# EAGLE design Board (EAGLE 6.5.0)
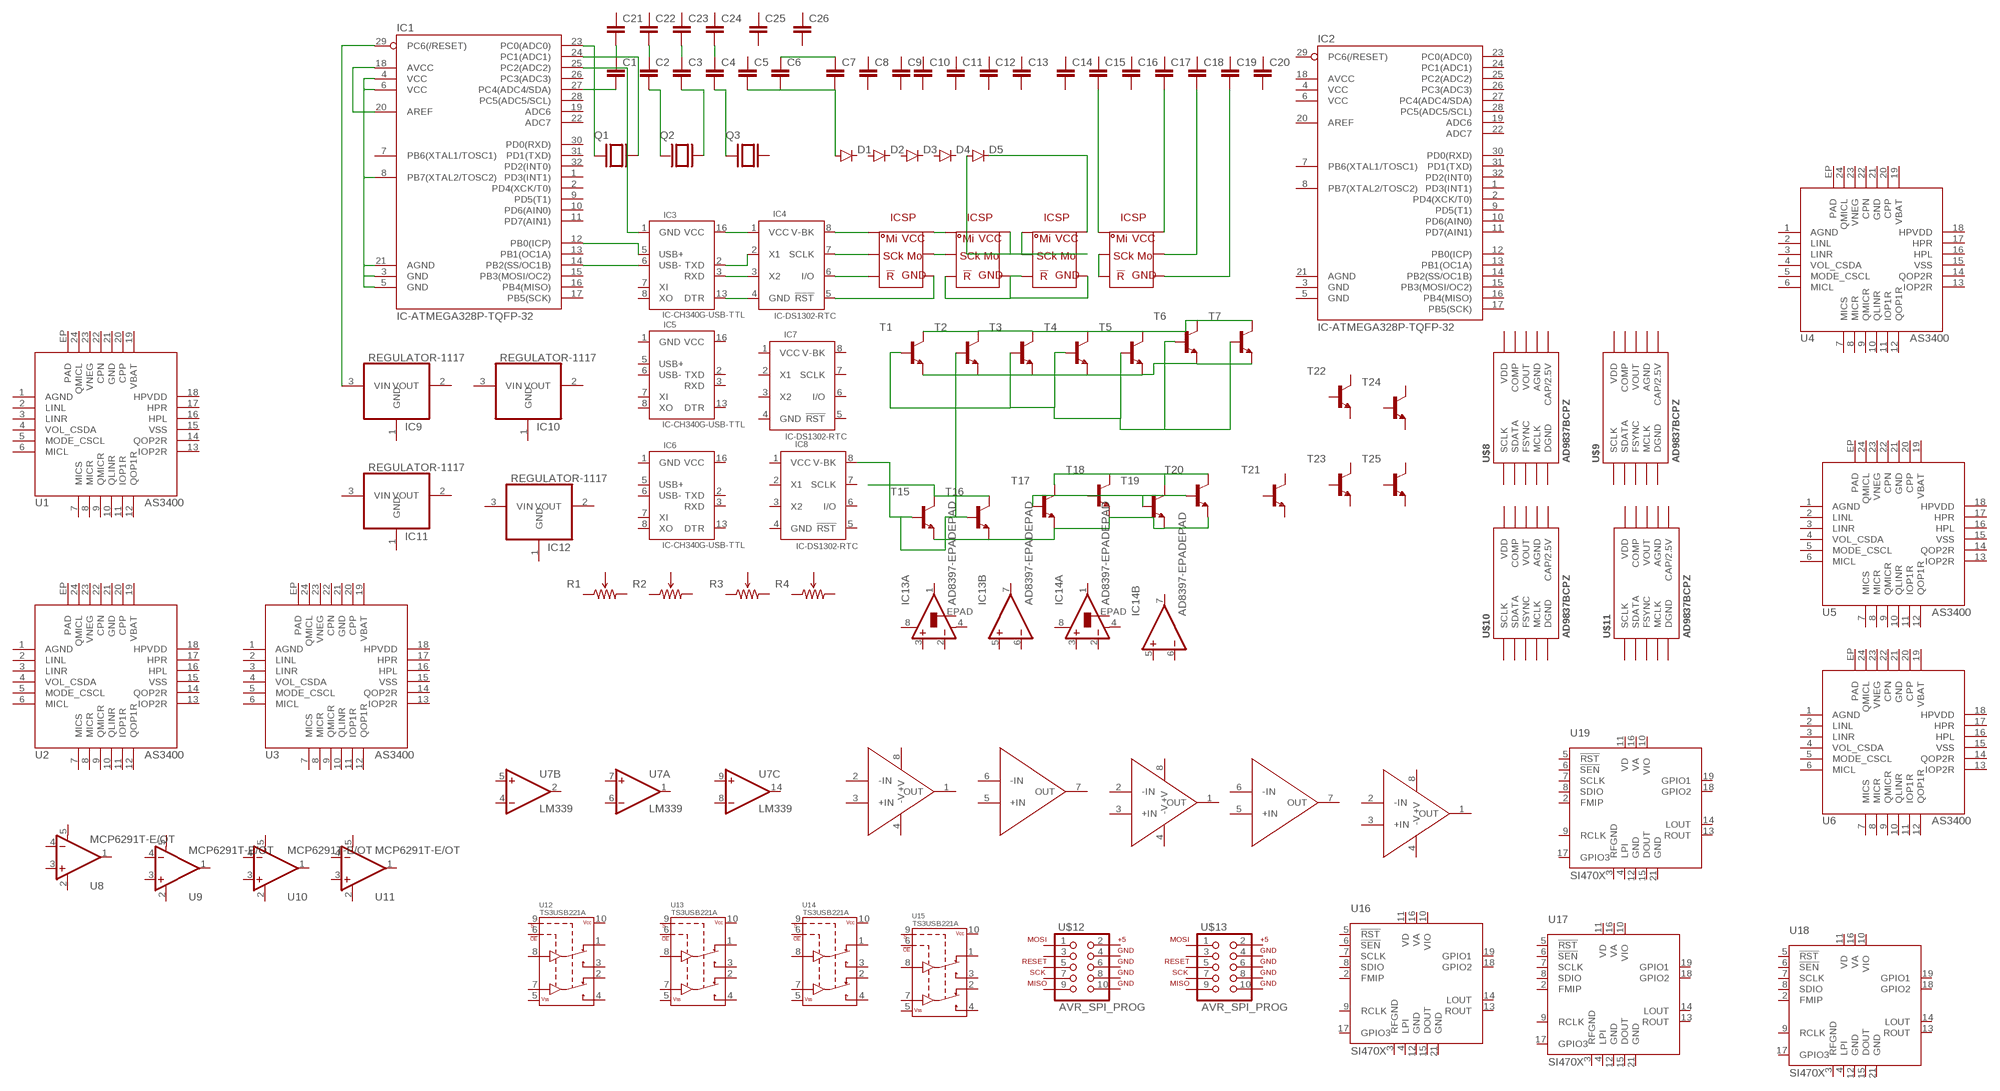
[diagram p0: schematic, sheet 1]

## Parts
C1  CAP-SMD-0603  [0603]
C2  CAP-SMD-0603  [0603]
C3  CAP-SMD-0603  [0603]
C4  CAP-SMD-0603  [0603]
C5  CAP-SMD-0603  [0603]
C6  CAP-SMD-0603  [0603]
C7  CAP-SMD-0805  [0805]
C8  CAP-SMD-0805  [0805]
C9  CAP-SMD-0805  [0805]
C10  CAP-SMD-0805  [0805]
C11  CAP-SMD-0805  [0805]
C12  CAP-SMD-0805  [0805]
C13  CAP-SMD-0805  [0805]
C14  CAP-SMD-1206  [1206]
C15  CAP-SMD-1206  [1206]
C16  CAP-SMD-1206  [1206]
C17  CAP-SMD-1206  [1206]
C18  CAP-SMD-1206  [1206]
C19  CAP-SMD-1206  [1206]
C20  CAP-SMD-1206  [1206]
C21  CAP-SMD-0603  [0603]
C22  CAP-SMD-0603  [0603]
C23  CAP-SMD-0603  [0603]
C24  CAP-SMD-0603  [0603]
C25  CAP-SMD-0603  [0603]
C26  CAP-SMD-0603  [0603]
D1  DIODE-SMA-4MM  [DIODE-SMA]
D2  DIODE-SMA-4MM  [DIODE-SMA]
D3  DIODE-SMA-4MM  [DIODE-SMA]
D4  DIODE-SMA-4MM  [DIODE-SMA]
D5  DIODE-SMA-4MM  [DIODE-SMA]
IC1  IC-ATMEGA328P-TQFP-32  [TQFP32-08MM]
IC2  IC-ATMEGA328P-TQFP-32  [TQFP32-08MM]
IC3  IC-CH340G-USB-TTL  [SOP-16]
IC4  IC-DS1302-RTC  [SOP-08]
IC5  IC-CH340G-USB-TTL  [SOP-16]
IC6  IC-CH340G-USB-TTL  [SOP-16]
IC7  IC-DS1302-RTC  [SOP-08]
IC8  IC-DS1302-RTC  [SOP-08]
IC9  REGULATOR-1117  [SOT-223]
IC10  REGULATOR-1117  [SOT-223]
IC11  REGULATOR-1117  [SOT-223]
IC12  REGULATOR-1117  [SOT-223]
IC13  AD8397-EPADEPAD  [SO08-EPAD]
IC14  AD8397-EPADEPAD  [SO08-EPAD]
Q1  CRYSTAL-5032  [CRYSTAL-5032]
Q2  CRYSTAL-5032  [CRYSTAL-5032]
Q3  CRYSTAL-5032  [CRYSTAL-5032]
R1  POTENTIOMETER-3MM-SMD  [POT-3MM-SMD]
R2  POTENTIOMETER-3MM-SMD  [POT-3MM-SMD]
R3  POTENTIOMETER-3MM-SMD  [POT-3MM-SMD]
R4  POTENTIOMETER-3MM-SMD  [POT-3MM-SMD]
T1  NPN-2SD882-D882-0.5W  [SOT-89]
T2  NPN-2SD882-D882-0.5W  [SOT-89]
T3  NPN-2SD882-D882-0.5W  [SOT-89]
T4  NPN-2SD882-D882-0.5W  [SOT-89]
T5  NPN-2SD882-D882-0.5W  [SOT-89]
T6  NPN-2SD882-D882-0.5W  [SOT-89]
T7  NPN-2SD882-D882-0.5W  [SOT-89]
T15  NPN-S9018-J8-0.2W  [SOT-23]
T16  NPN-S9018-J8-0.2W  [SOT-23]
T17  NPN-S9018-J8-0.2W  [SOT-23]
T18  NPN-S9018-J8-0.2W  [SOT-23]
T19  NPN-S9018-J8-0.2W  [SOT-23]
T20  NPN-S9018-J8-0.2W  [SOT-23]
T21  NPN-S9018-J8-0.2W  [SOT-23]
T22  NPN-TO-92  [TO-92]
T23  NPN-TO-92  [TO-92]
T24  NPN-TO-92  [TO-92]
T25  NPN-TO-92  [TO-92]
U1  AS3400  [QFN-24_ALT2]
U2  AS3400  [QFN-24_ALT2]
U3  AS3400  [QFN-24_ALT2]
U4  AS3400  [QFN-24_ALT2]
U5  AS3400  [QFN-24_ALT2]
U6  AS3400  [QFN-24_ALT2]
U7  LM339  [TSSOP-14]
U8  MCP6291T-E/OT  [SOT23-5]
U9  MCP6291T-E/OT  [SOT23-5]
U10  MCP6291T-E/OT  [SOT23-5]
U11  MCP6291T-E/OT  [SOT23-5]
U12  TS3USB221A  [QFN-10-RSE]
U13  TS3USB221A  [QFN-10-RSE]
U14  TS3USB221A  [QFN-10-RSE]
U15  TS3USB221A  [QFN-10-RSE]
U16  SI470X  [SI470X]
U17  SI470X  [SI470X]
U18  SI470X  [SI470X]
U19  SI470X  [SI470X]
U$1  ISCP-6PINS  [ISCP]
U$2  ISCP-6PINS  [ISCP]
U$3  ISCP-6PINS  [ISCP]
U$4  ISCP-6PINS  [ISCP]
U$5  LTC6244  [MSOP8]
U$6  LTC6244  [MSOP8]
U$7  LTC6244  [MSOP8]
U$8  AD9837BCPZ  AD9837  [AD9837]
U$9  AD9837BCPZ  AD9837  [AD9837]
U$10  AD9837BCPZ  AD9837  [AD9837]
U$11  AD9837BCPZ  AD9837  [AD9837]
U$12  AVR_SPI_PROG  [AVR_ICSP]
U$13  AVR_SPI_PROG  [AVR_ICSP]

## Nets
N$27: IC1.29(PC6(/RESET)) IC9.3(VIN)
N$28: IC1.18(AVCC) IC1.20(AREF)
N$29: IC1.6(VCC) IC1.8(PB7(XTAL2/TOSC2))
N$30: IC1.3(GND) IC1.4(VCC) IC1.5(GND) IC1.21(AGND)
N$31: IC1.23(PC0(ADC0)) Q1.1
N$32: C21.2 IC1.24(PC1(ADC1)) Q1.2
N$33: C6.1 C7.1
N$34: C5.2 D1.A
N$35: C4.2 Q3.1
N$36: C3.2 Q2.2
N$37: C2.2 Q2.1
N$38: C4.1 C24.2
N$39: C3.1 C23.2
N$40: C2.1 C22.2
N$41: C1.2 IC1.27(PC4(ADC4/SDA))
N$42: IC1.25(PC2(ADC2)) IC3.1(GND)
N$43: IC1.12(PB0(ICP)) IC3.5(USB+)
N$44: IC1.14(PB2(SS/OC1B)) IC3.6(USB-)
N$45: IC3.16(VCC) IC4.1(VCC)
N$46: IC3.3(RXD) IC4.3(X2)
N$47: IC3.2(TXD) IC4.2(X1)
N$48: IC3.13(DTR) IC4.4(GND)
N$49: IC4.8(V-BK) U$1.P$1
N$50: IC4.7(SCLK) U$1.P$2
N$51: IC4.6(I/O) U$1.P$3
N$52: IC4.5(!RST) U$1.P$4
N$53: U$1.P$5 U$2.P$2
N$54: U$1.P$6 U$2.P$1
N$55: U$2.P$3 U$2.P$4 U$3.P$3 U$3.P$4
N$56: U$2.P$5 U$2.P$6
N$57: U$3.P$1 U$3.P$2
N$59: D5.C U$3.P$6
N$60: C15.2 U$4.P$1
N$61: D5.A U$3.P$5
N$62: U$4.P$2 U$4.P$3
N$63: C17.2 U$4.P$6
N$64: C18.2 U$4.P$5
N$65: C19.2 U$4.P$4
N$66: IC8.8(V-BK) T15.1(B) T16.1(B)
N$67: T15.3(C) T16.3(C)
N$68: T2.1(B)
N$69: T1.1(B) T3.1(B) T4.1(B) T5.1(B) T6.1(B) T7.1(B)
N$74: T1.2(C) T2.2(C) T3.2(C) T4.2(C) T5.2(C) T6.2(C) T7.2(C)
N$75: T1.3(E) T2.3(E) T3.3(E) T4.3(E) T5.3(E) T6.3(E) T7.3(E)
N$78: T15.2(E) T16.2(E) T17.2(E) T18.2(E) T19.2(E) T20.2(E)
N$81: T17.3(C) T18.3(C) T19.3(C) T20.3(C)
N$82: T17.1(B) T18.1(B) T19.1(B) T20.1(B)
Unconnected: C1.1 C5.1 C6.2 C7.2 C8.1 C8.2 C9.1 C9.2 C10.1 C10.2 C11.1 C11.2 C12.1 C12.2 C13.1 C13.2 C14.1 C14.2 C15.1 C16.1 C16.2 C17.1 C18.1 C19.1 C20.1 C20.2 C21.1 C22.1 C23.1 C24.1 C25.1 C25.2 C26.1 C26.2 D1.C D2.A D2.C D3.A D3.C D4.A D4.C IC1.1(PD3(INT1)) IC1.2(PD4(XCK/T0)) IC1.7(PB6(XTAL1/TOSC1)) IC1.9(PD5(T1)) IC1.10(PD6(AIN0)) IC1.11(PD7(AIN1)) IC1.13(PB1(OC1A)) IC1.15(PB3(MOSI/OC2)) IC1.16(PB4(MISO)) IC1.17(PB5(SCK)) IC1.19(ADC6) IC1.22(ADC7) IC1.26(PC3(ADC3)) IC1.28(PC5(ADC5/SCL)) IC1.30(PD0(RXD)) IC1.31(PD1(TXD)) IC1.32(PD2(INT0)) IC2.1(PD3(INT1)) IC2.2(PD4(XCK/T0)) IC2.3(GND) IC2.4(VCC) IC2.5(GND) IC2.6(VCC) IC2.7(PB6(XTAL1/TOSC1)) IC2.8(PB7(XTAL2/TOSC2)) IC2.9(PD5(T1)) IC2.10(PD6(AIN0)) IC2.11(PD7(AIN1)) IC2.12(PB0(ICP)) IC2.13(PB1(OC1A)) IC2.14(PB2(SS/OC1B)) IC2.15(PB3(MOSI/OC2)) IC2.16(PB4(MISO)) IC2.17(PB5(SCK)) IC2.18(AVCC) IC2.19(ADC6) IC2.20(AREF) IC2.21(AGND) IC2.22(ADC7) IC2.23(PC0(ADC0)) IC2.24(PC1(ADC1)) IC2.25(PC2(ADC2)) IC2.26(PC3(ADC3)) IC2.27(PC4(ADC4/SDA)) IC2.28(PC5(ADC5/SCL)) IC2.29(PC6(/RESET)) IC2.30(PD0(RXD)) IC2.31(PD1(TXD)) IC2.32(PD2(INT0)) IC3.7(XI) IC3.8(XO) IC5.1(GND) IC5.2(TXD) IC5.3(RXD) IC5.5(USB+) IC5.6(USB-) IC5.7(XI) IC5.8(XO) IC5.13(DTR) IC5.16(VCC) IC6.1(GND) IC6.2(TXD) IC6.3(RXD) IC6.5(USB+) IC6.6(USB-) IC6.7(XI) IC6.8(XO) IC6.13(DTR) IC6.16(VCC) IC7.1(VCC) IC7.2(X1) IC7.3(X2) IC7.4(GND) IC7.5(!RST) IC7.6(I/O) IC7.7(SCLK) IC7.8(V-BK) IC8.1(VCC) IC8.2(X1) IC8.3(X2) IC8.4(GND) IC8.5(!RST) IC8.6(I/O) IC8.7(SCLK) IC9.2(VOUT) IC10.2(VOUT) IC10.3(VIN) IC11.2(VOUT) IC11.3(VIN) IC12.2(VOUT) IC12.3(VIN) IC13.1(A:OUT) IC13.2(A:-IN) IC13.3(A:+IN) IC13.5(B:+IN) IC13.6(B:-IN) IC13.7(B:OUT) IC13.EPAD(A:EPAD) IC14.1(A:OUT) IC14.2(A:-IN) IC14.3(A:+IN) IC14.5(B:+IN) IC14.6(B:-IN) IC14.7(B:OUT) IC14.EPAD(A:EPAD) Q3.2 R1.1(CCW) R1.2(WIPER) R1.3(CW) R2.1(CCW) R2.2(WIPER) R2.3(CW) R3.1(CCW) R3.2(WIPER) R3.3(CW) R4.1(CCW) R4.2(WIPER) R4.3(CW) T21.1(B) T21.2(E) T21.3(C) T22.1(E) T22.2(B) T22.3(C) T23.1(E) T23.2(B) T23.3(C) T24.1(E) T24.2(B) T24.3(C) T25.1(E) T25.2(B) T25.3(C) U1.1(AGND) U1.2(LINL) U1.3(LINR) U1.4(VOL_CSDA) U1.5(MODE_CSCL) U1.6(MICL) U1.7(MICS) U1.8(MICR) U1.9(QMICR) U1.10(QLINR) U1.11(IOP1R) U1.12(QOP1R) U1.13(IOP2R) U1.14(QOP2R) U1.15(VSS) U1.16(HPL) U1.17(HPR) U1.18(HPVDD) U1.19(VBAT) U1.20(CPP) U1.21(GND) U1.22(CPN) U1.23(VNEG) U1.24(QMICL) U1.EP(PAD) U2.1(AGND) U2.2(LINL) U2.3(LINR) U2.4(VOL_CSDA) U2.5(MODE_CSCL) U2.6(MICL) U2.7(MICS) U2.8(MICR) U2.9(QMICR) U2.10(QLINR) U2.11(IOP1R) U2.12(QOP1R) U2.13(IOP2R) U2.14(QOP2R) U2.15(VSS) U2.16(HPL) U2.17(HPR) U2.18(HPVDD) U2.19(VBAT) U2.20(CPP) U2.21(GND) U2.22(CPN) U2.23(VNEG) U2.24(QMICL) U2.EP(PAD) U3.1(AGND) U3.2(LINL) U3.3(LINR) U3.4(VOL_CSDA) U3.5(MODE_CSCL) U3.6(MICL) U3.7(MICS) U3.8(MICR) U3.9(QMICR) U3.10(QLINR) U3.11(IOP1R) U3.12(QOP1R) U3.13(IOP2R) U3.14(QOP2R) U3.15(VSS) U3.16(HPL) U3.17(HPR) U3.18(HPVDD) U3.19(VBAT) U3.20(CPP) U3.21(GND) U3.22(CPN) U3.23(VNEG) U3.24(QMICL) U3.EP(PAD) U4.1(AGND) U4.2(LINL) U4.3(LINR) U4.4(VOL_CSDA) U4.5(MODE_CSCL) U4.6(MICL) U4.7(MICS) U4.8(MICR) U4.9(QMICR) U4.10(QLINR) U4.11(IOP1R) U4.12(QOP1R) U4.13(IOP2R) U4.14(QOP2R) U4.15(VSS) U4.16(HPL) U4.17(HPR) U4.18(HPVDD) U4.19(VBAT) U4.20(CPP) U4.21(GND) U4.22(CPN) U4.23(VNEG) U4.24(QMICL) U4.EP(PAD) U5.1(AGND) U5.2(LINL) U5.3(LINR) U5.4(VOL_CSDA) U5.5(MODE_CSCL) U5.6(MICL) U5.7(MICS) U5.8(MICR) U5.9(QMICR) U5.10(QLINR) U5.11(IOP1R) U5.12(QOP1R) U5.13(IOP2R) U5.14(QOP2R) U5.15(VSS) U5.16(HPL) U5.17(HPR) U5.18(HPVDD) U5.19(VBAT) U5.20(CPP) U5.21(GND) U5.22(CPN) U5.23(VNEG) U5.24(QMICL) U5.EP(PAD) U6.1(AGND) U6.2(LINL) U6.3(LINR) U6.4(VOL_CSDA) U6.5(MODE_CSCL) U6.6(MICL) U6.7(MICS) U6.8(MICR) U6.9(QMICR) U6.10(QLINR) U6.11(IOP1R) U6.12(QOP1R) U6.13(IOP2R) U6.14(QOP2R) U6.15(VSS) U6.16(HPL) U6.17(HPR) U6.18(HPVDD) U6.19(VBAT) U6.20(CPP) U6.21(GND) U6.22(CPN) U6.23(VNEG) U6.24(QMICL) U6.EP(PAD) U7.1(A:OUT) U7.2(B:OUT) U7.4(B:-IN) U7.5(B:+IN) U7.6(A:-IN) U7.7(A:+IN) U7.8(C:-IN) U7.9(C:+IN) U7.10(D:-IN) U7.11(D:+IN) U7.13(D:OUT) U7.14(C:OUT) U8.1(OUT) U8.3(+IN) U8.4(-IN) U9.1(OUT) U9.3(+IN) U9.4(-IN) U10.1(OUT) U10.3(+IN) U10.4(-IN) U11.1(OUT) U11.3(+IN) U11.4(-IN) U12.1(1D+) U12.2(1D-) U12.3(2D+) U12.4(2D-) U12.5(VSS) U12.6(!OE) U12.7(D-) U12.8(D+) U12.9(S) U12.10(VCC) U13.1(1D+) U13.2(1D-) U13.3(2D+) U13.4(2D-) U13.5(VSS) U13.6(!OE) U13.7(D-) U13.8(D+) U13.9(S) U13.10(VCC) U14.1(1D+) U14.2(1D-) U14.3(2D+) U14.4(2D-) U14.5(VSS) U14.6(!OE) U14.7(D-) U14.8(D+) U14.9(S) U14.10(VCC) U15.1(1D+) U15.2(1D-) U15.3(2D+) U15.4(2D-) U15.5(VSS) U15.6(!OE) U15.7(D-) U15.8(D+) U15.9(S) U15.10(VCC) U16.2(FMIP) U16.3(RFGND) U16.4(LPI) U16.5(!RST) U16.6(!SEN) U16.7(SCLK) U16.8(SDIO) U16.9(RCLK) U16.10(VIO) U16.11(VD) U16.12(GND) U16.13(ROUT) U16.14(LOUT) U16.15(DOUT) U16.16(VA) U16.17(GPIO3) U16.18(GPIO2) U16.19(GPIO1) U16.21(GND) U17.2(FMIP) U17.3(RFGND) U17.4(LPI) U17.5(!RST) U17.6(!SEN) U17.7(SCLK) U17.8(SDIO) U17.9(RCLK) U17.10(VIO) U17.11(VD) U17.12(GND) U17.13(ROUT) U17.14(LOUT) U17.15(DOUT) U17.16(VA) U17.17(GPIO3) U17.18(GPIO2) U17.19(GPIO1) U17.21(GND) U18.2(FMIP) U18.3(RFGND) U18.4(LPI) U18.5(!RST) U18.6(!SEN) U18.7(SCLK) U18.8(SDIO) U18.9(RCLK) U18.10(VIO) U18.11(VD) U18.12(GND) U18.13(ROUT) U18.14(LOUT) U18.15(DOUT) U18.16(VA) U18.17(GPIO3) U18.18(GPIO2) U18.19(GPIO1) U18.21(GND) U19.2(FMIP) U19.3(RFGND) U19.4(LPI) U19.5(!RST) U19.6(!SEN) U19.7(SCLK) U19.8(SDIO) U19.9(RCLK) U19.10(VIO) U19.11(VD) U19.12(GND) U19.13(ROUT) U19.14(LOUT) U19.15(DOUT) U19.16(VA) U19.17(GPIO3) U19.18(GPIO2) U19.19(GPIO1) U19.21(GND) U$5.1(OUT) U$5.2(-IN) U$5.3(+IN) U$5.4(-V) U$5.5(+IN) U$5.6(-IN) U$5.7(OUT) U$5.8(+V) U$6.1(OUT) U$6.2(-IN) U$6.3(+IN) U$6.4(-V) U$6.5(+IN) U$6.6(-IN) U$6.7(OUT) U$6.8(+V) U$7.1(OUT) U$7.2(-IN) U$7.3(+IN) U$7.4(-V) U$7.5(+IN) U$7.6(-IN) U$7.7(OUT) U$7.8(+V) U$8.P$0(DGND) U$8.P$1(COMP) U$8.P$2(VDD) U$8.P$3(CAP/2.5V) U$8.P$4(DGND) U$8.P$5(MCLK) U$8.P$6(SDATA) U$8.P$7(SCLK) U$8.P$8(FSYNC) U$8.P$9(AGND) U$8.P$10(VOUT) U$9.P$0(DGND) U$9.P$1(COMP) U$9.P$2(VDD) U$9.P$3(CAP/2.5V) U$9.P$4(DGND) U$9.P$5(MCLK) U$9.P$6(SDATA) U$9.P$7(SCLK) U$9.P$8(FSYNC) U$9.P$9(AGND) U$9.P$10(VOUT) U$10.P$0(DGND) U$10.P$1(COMP) U$10.P$2(VDD) U$10.P$3(CAP/2.5V) U$10.P$4(DGND) U$10.P$5(MCLK) U$10.P$6(SDATA) U$10.P$7(SCLK) U$10.P$8(FSYNC) U$10.P$9(AGND) U$10.P$10(VOUT) U$11.P$0(DGND) U$11.P$1(COMP) U$11.P$2(VDD) U$11.P$3(CAP/2.5V) U$11.P$4(DGND) U$11.P$5(MCLK) U$11.P$6(SDATA) U$11.P$7(SCLK) U$11.P$8(FSYNC) U$11.P$9(AGND) U$11.P$10(VOUT) U$12.1 U$12.2 U$12.3 U$12.4 U$12.5 U$12.6 U$12.7 U$12.8 U$12.9 U$12.10 U$13.1 U$13.2 U$13.3 U$13.4 U$13.5 U$13.6 U$13.7 U$13.8 U$13.9 U$13.10

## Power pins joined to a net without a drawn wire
GND: IC9.1(GND) IC10.1(GND) IC11.1(GND) IC12.1(GND) U7.12(P:GND)
V+: IC13.8(A:V+) IC14.8(A:V+) U8.5(V+) U9.5(V+) U10.5(V+) U11.5(V+)
V-: IC13.4(A:V-) IC14.4(A:V-) U8.2(V-) U9.2(V-) U10.2(V-) U11.2(V-)
VCC: U7.3(P:VCC)

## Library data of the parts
C1-C26 = - Jins eagle lbr:CAP-SMD
D1-D5 = - Jins eagle lbr:DIODE: Diode
IC1 IC2 = - Jins eagle lbr:IC-ATMEGA328P-TQFP-32
IC3 IC5 IC6 = - Jins eagle lbr:IC-CH340G
IC4 IC7 IC8 = - Jins eagle lbr:IC-DS1302
IC9-IC12 = - Jins eagle lbr:REGULATOR: 800mA and 1A Low Dropout (LDO) Positive Regulator 1.8V, 2.5V, 2.85V, 3.3V, 5V, and Adj; MPN: REG1117; OC_FARNELL: 1097566; OC_NEWARK: 14P6981
IC13 IC14 = SparkFun-AnalogIC:AD8397-EPAD: Rail-to-rail high current output op-amp
Q1-Q3 = - Jins eagle lbr:CRYSTAL: CRYSTAL
R1-R4 = - Jins eagle lbr:POTENTIOMETER
T1-T7 T15-T25 = - Jins eagle lbr:NPN
U1-U6 = SparkFun-AnalogIC:AS3400: Active noise cancellation chip. Stereo in, stereo out, two microphones. Single alkaline cell power. QFN-24 w/exposed pad.
U7 = SparkFun-AnalogIC:LM339: Based on information from the SLCS006N datasheet from TI (www.ti.com). Change Log DateAuthorChange July 16, 2008nick@scantool.netDevice created.; DESC: IC, Quad Comparator; MANUF: Texas Instruments; PARTNUM: LM339PWR; SUPPLIER: Digikey:296-6607-1-ND; VALSTAT: PARTNUM
U8-U11 = SparkFun-AnalogIC:MCP6291: Rail to rail OpAmp with 10MHz GBP; PROD_ID: IC-11991
U12-U15 = SparkFun-AnalogIC:TS3USB221A: DPDT Analog Mux Vcc 2.5 to 3.3V Passes up to 5.5V at 3.3V supply 900MHz BW, 6&#8486; switch resistance; PROD_ID: IC-12115
U16-U19 = SparkFun-RF:SI470X: FM receiver IC. Tested with Si4703. You really only need SEN, RST, SCLK, and SDIO to get a full FM radio working. Antenna comes from headphone jack. See BOB-10344.
U$1-U$4 = - Jins eagle lbr:ISCP
U$5-U$7 = SparkFun-AnalogIC:LTC6244: Low-noise, high-speed rail-to-rail CMOS op-amp
U$8-U$11 = SparkFun-AnalogIC:AD9837: Programmable waveform generator, sine, triangular, and square wave outputs.; PROD_ID: IC-11223
U$12 U$13 = SparkFun-Connectors:AVR_SPI_PROG: AVR 10-pin ICSP Header This is the standard AVR In Circuit Serial Programming header. Minimal, but includes pin one indicator. Works with standard Olimex programmers. Also look for the 6-pin reduced version. Spark Fun Electronics SKU: PRT-00778

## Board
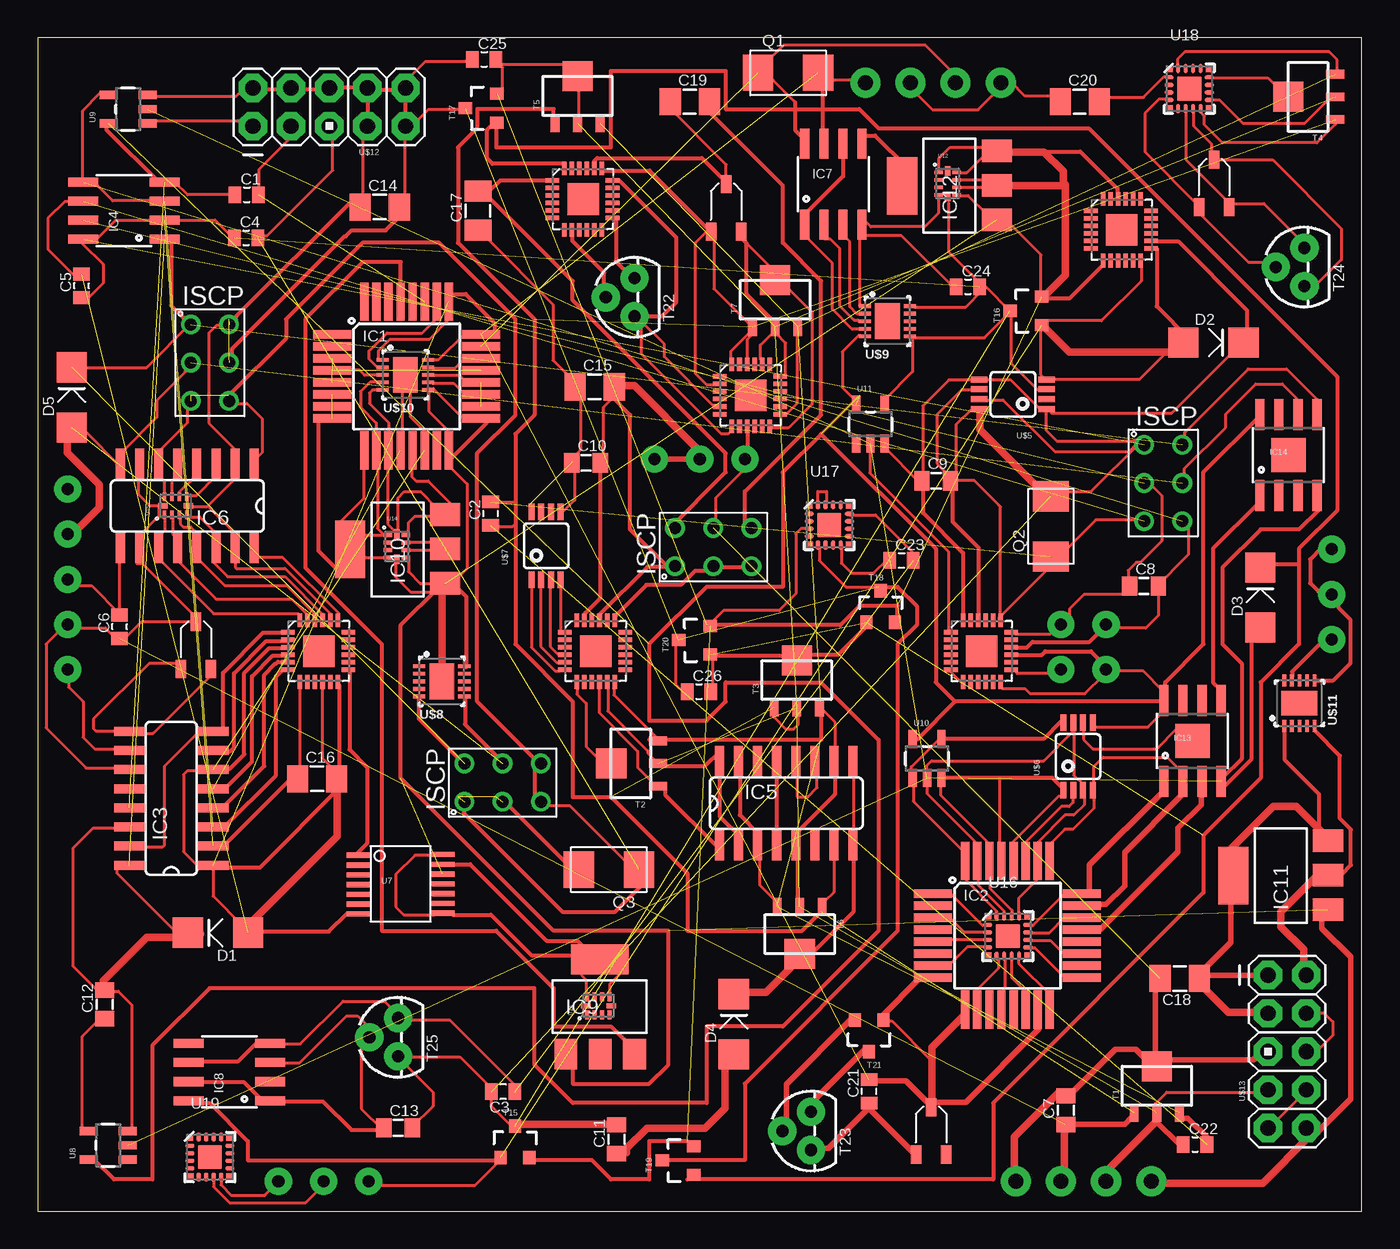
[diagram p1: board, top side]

Size 88 x 78 mm. Coordinates in mm from the lower left corner, seen from the top.
Outline: 0,0 88,0 88,78 0,78 0,0
Copper layers (1*16): Top 0.035mm / dielectric 1.5mm / Bottom 0.035mm
Design rules "default": minimum track width 10mil, minimum drill 24mil, track to track 8mil, track to pad 8mil, pad to pad 8mil, via to via 8mil, smd to smd 8mil, copper to edge 40mil, drill to drill 8mil, minimum pad ring 10mil, minimum via ring 8mil, stop-mask expansion 4mil, vias tented up to drill 0mil, thermal gap 10mil

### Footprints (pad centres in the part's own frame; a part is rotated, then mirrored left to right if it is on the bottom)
0603 = smd 0.838 x 1.1: 1 -0.781,0; 2 0.781,0
0805 = smd 1.016 x 1.27: 1 -0.95,0; 2 0.95,0
1206 = smd 1.4 x 1.8: 1 -1.3,0; 2 1.3,0
DIODE-SMA = smd 2 x 2: A -2,0; C 2,0
TQFP32-08MM = smd 2.54 x 0.559: 1 -6.502,6.75; 2 -6.502,5.95; 3 -6.502,5.15; 4 -6.502,4.35; 5 -6.502,3.55; 6 -6.502,2.75; 7 -6.502,1.95; 8 -6.502,1.15; 17 3.404,1.15; 18 3.404,1.95; 19 3.404,2.75; 20 3.404,3.55; 21 3.404,4.35; 22 3.404,5.15; 23 3.404,5.95; 24 3.404,6.75 | smd 0.559 x 2.54: 9 -4.35,-0.965; 10 -3.55,-0.965; 11 -2.75,-0.965; 12 -1.95,-0.965; 13 -1.15,-0.965; 14 -0.35,-0.965; 15 0.45,-0.965; 16 1.25,-0.965; 25 1.25,8.915; 26 0.45,8.915; 27 -0.35,8.915; 28 -1.15,8.915; 29 -1.95,8.915; 30 -2.75,8.915; 31 -3.55,8.915; 32 -4.35,8.915
SOP-16 = smd 0.6 x 2: 1 -3.945,-2.76; 2 -2.675,-2.76; 3 -1.405,-2.76; 4 -0.135,-2.76; 5 1.135,-2.76; 6 2.405,-2.76; 7 3.675,-2.76; 8 4.945,-2.76; 9 4.945,2.84; 10 3.675,2.84; 11 2.405,2.84; 12 1.135,2.84; 13 -0.135,2.84; 14 -1.405,2.84; 15 -2.675,2.84; 16 -3.945,2.84
SOP-08 = smd 0.6 x 2: 1 -1.905,-2.7; 2 -0.635,-2.7; 3 0.635,-2.7; 4 1.905,-2.7; 5 1.905,2.7; 6 0.635,2.7; 7 -0.635,2.7; 8 -1.905,2.7
SOT-223 = smd 1.499 x 2.007: 1 -2.261,-3.15; 2 0.025,-3.15; 3 2.311,-3.15 | smd 3.81 x 2.007: 4 0,3.15
SO08-EPAD = smd 0.61 x 2.057: 1 -1.905,-2.692; 2 -0.635,-2.692; 3 0.635,-2.692; 4 1.905,-2.692; 5 1.905,2.692; 6 0.635,2.692; 7 -0.635,2.692; 8 -1.905,2.692 | smd 2.286 x 2.286: EPAD 0,0
CRYSTAL-5032 = smd 2 x 2.4: 1 -2,0; 2 2,0
POT-3MM-SMD = smd 0.7 x 1.2: 1 -1,-1.55; 2 0,1.6; 3 1,-1.55
SOT-89 = smd 0.58 x 1.2: 1 -1.5,-1.8; 2 0,-1.8; 3 1.5,-1.8 | smd 2 x 2: 4 0,1.3
SOT-23 = smd 0.8 x 0.9: 1 -1.315,-0.635; 2 0.585,-0.635; 3 -0.365,1.465
TO-92 = drill 0.813 pad 1.88: 1 -1.27,0; 2 0,1.905; 3 1.27,0
QFN-24_ALT2 = smd 0.9 x 0.3: 1 -2.05,1.25; 2 -2.05,0.75; 3 -2.05,0.25; 4 -2.05,-0.25; 5 -2.05,-0.75; 6 -2.05,-1.25; 13 1.95,-1.25; 14 1.95,-0.75; 15 1.95,-0.25; 16 1.95,0.25; 17 1.95,0.75; 18 1.95,1.25 | smd 0.3 x 0.9: 7 -1.25,-2.05; 8 -0.75,-2.05; 9 -0.25,-2.05; 10 0.25,-2.05; 11 0.75,-2.05; 12 1.25,-2.05; 19 1.25,2.05; 20 0.75,2.05; 21 0.25,2.05; 22 -0.25,2.05; 23 -0.75,2.05; 24 -1.25,2.05 | smd 2.1 x 2.1: EP 0,0
TSSOP-14 = smd 1.6 x 0.35: 1 -2.8,1.9; 2 -2.8,1.25; 3 -2.8,0.6; 4 -2.8,-0.05; 5 -2.8,-0.7; 6 -2.8,-1.35; 7 -2.8,-2; 8 2.8,-1.95; 9 2.8,-1.3; 10 2.8,-0.65; 11 2.8,0; 12 2.8,0.65; 13 2.8,1.3; 14 2.8,1.95
SOT23-5 = smd 0.55 x 1.2: 1 -0.95,-1.3; 2 0,-1.3; 3 0.95,-1.3; 4 0.95,1.3; 5 -0.95,1.3
QFN-10-RSE = smd 0.58 x 0.25: 1 -0.6,0.75; 2 -0.6,0.25; 3 -0.6,-0.25; 4 -0.6,-0.75; 6 0.6,-0.75; 7 0.6,-0.25; 8 0.6,0.25; 9 0.6,0.75 | smd 0.35 x 0.63: 5 0,-0.85; 10 0,0.85
SI470X = smd 0.34 x 0.34: 1 -1.275,1.265; 6 -1.265,-1.265; 11 1.265,-1.265; 16 1.265,1.265 | smd 0.61 x 0.28: 2 -1.335,0.75; 3 -1.335,0.25; 4 -1.335,-0.25; 5 -1.335,-0.75; 12 1.335,-0.75; 13 1.335,-0.25; 14 1.335,0.25; 15 1.335,0.75 | smd 0.28 x 0.61: 7 -0.75,-1.335; 8 -0.25,-1.335; 9 0.25,-1.335; 10 0.75,-1.335; 17 0.75,1.335; 18 0.25,1.335; 19 -0.25,1.335; 20 -0.75,1.335 | smd 1.6 x 1.6: 21 0,0
ISCP = drill 0.8: P$1 -2.54,2.54; P$2 -2.54,0; P$3 -2.54,-2.54; P$4 0,-2.54; P$5 0,0; P$6 0,2.54
MSOP8 = smd 0.4 x 1.1: 1 -0.975,-2.25; 2 -0.325,-2.25; 3 0.325,-2.25; 4 0.975,-2.25; 5 0.975,2.25; 6 0.325,2.25; 7 -0.325,2.25; 8 -0.975,2.25
AD9837 = smd 1.64 x 2.38: P$0 0,0 | smd 0.8 x 0.25: P$1 -1.5,1; P$2 -1.5,0.5; P$3 -1.5,0; P$4 -1.5,-0.5; P$5 -1.5,-1; P$6 1.5,-1; P$7 1.5,-0.5; P$8 1.5,0; P$9 1.5,0.5; P$10 1.5,1
AVR_ICSP = drill 1.016 pad 1.88 octagon: 1 -1.27,5.08; 2 1.27,5.08; 3 -1.27,2.54; 4 1.27,2.54; 5 -1.27,0; 6 1.27,0; 7 -1.27,-2.54; 8 1.27,-2.54; 9 -1.27,-5.08; 10 1.27,-5.08

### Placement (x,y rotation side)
C1  13.9,67.55 0 top
C2  30.1,46.37 90 top
C3  30.94,7.96 180 top
C4  13.85,64.7 0 top
C5  2.92,61.5 90 top
C6  5.45,38.85 90 top
C7  68.33,6.72 90 top
C8  73.52,41.55 0 top
C9  59.71,48.55 0 top
C10  36.45,49.74 0 top
C11  38.47,4.8 90 top
C12  4.45,13.76 90 top
C13  23.95,5.55 0 top
C14  22.74,66.74 0 top
C15  37.02,54.79 0 top
C16  18.58,28.74 0 top
C17  29.26,66.5 90 top
C18  75.89,15.48 180 top
C19  43.34,73.74 0 top
C20  69.26,73.74 0 top
C21  55.24,7.97 90 top
C22  76.91,4.44 0 top
C23  57.4,43.25 0 top
C24  61.82,61.44 0 top
C25  29.67,76.55 0 top
C26  43.94,34.54 0 top
D1  11.99,18.52 180 top
D2  78.14,57.74 0 top
D3  81.26,40.79 90 top
D4  46.26,12.44 90 top
D5  2.26,54.09 90 top
IC1  26.07,51.54 0 top
IC2  66,14.37 0 top
IC3  8.92,26.95 90 top
IC4  5.74,66.5 90 top
IC5  49.25,27.08 0 top
IC6  10.45,46.92 180 top
IC7  52.88,68.26 0 top
IC8  12.74,9.26 90 top
IC9  37.35,13.6 0 top
IC10  23.92,44 90 top
IC11  82.6,22.31 90 top
IC12  60.6,68.15 90 top
IC13  76.74,31.26 0 top
IC14  83.12,50.26 0 top
Q1  49.87,75.66 0 top
Q2  67.34,45.52 90 top
Q3  37.96,22.71 180 top
R1  10.53,37.58 0 top
R2  59.38,5.33 0 top
R3  45.76,66.66 0 top
R4  78.17,68.29 0 top
T1  74.37,8.34 0 top
T2  39.42,29.76 90 top
T3  50.45,35.3 0 top
T4  84.42,74.06 90 top
T5  35.88,74.12 0 top
T6  50.64,18.42 180 top
T7  49.01,60.58 0 top
T15  32.09,4.21 0 top
T16  66.09,60.21 90 top
T17  29.89,73.67 90 top
T18  56.39,39.77 0 top
T19  42.96,3.75 90 top
T20  44.07,38.32 90 top
T21  54.89,12.08 180 top
T22  39.66,60.75 90 top
T23  51.39,5.34 90 top
T24  84.18,62.75 90 top
T25  23.95,11.57 90 top
U1  36.25,67.26 0 top
U2  37.09,37.23 0 top
U3  62.74,37.23 0 top
U4  47.39,54.23 0 top
U5  72.04,65.23 0 top
U6  18.69,37.23 0 top
U7  24.12,21.76 0 top
U8  4.69,4.39 90 top
U9  6.01,73.24 90 top
U10  59.11,30.09 0 top
U11  55.34,52.31 0 top
U12  60.47,68.3 0 top
U13  37.26,13.66 90 top
U14  23.88,44.19 0 top
U15  9.18,46.89 90 top
U16  64.47,18.29 0 top
U17  52.61,45.61 0 top
U18  76.53,74.61 0 top
U19  11.45,3.61 0 top
U$1  76.07,48.4 0 top
U$2  12.72,56.4 0 top
U$3  30.9,29.76 90 top
U$4  44.9,45.41 90 top
U$5  64.81,54.3 90 top
U$6  69.14,30.23 0 top
U$7  33.79,44.23 0 top
U$8  26.85,35.22 0 top
U$9  56.47,59.15 0 top
U$10  24.44,55.59 0 top
U$11  83.85,33.77 90 top
U$12  19.38,73.39 90 top
U$13  83.04,10.62 0 top

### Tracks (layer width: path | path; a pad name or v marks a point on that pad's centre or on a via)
GND  (3 unrouted)
  Top 0.254: IC10.1 26.67,41.5 24.13,38.96 24.13,28.8 34.29,18.64 41.91,18.64 41.91,9.75 40.64,8.48 35.56,8.48 35.56,9.75 IC9.1
N$1  (via drill 0.8 pad 1.8)
  other vias: 2,36
N$2  (via drill 0.8 pad 1.8)
  other vias: 2,45
N$3  (via drill 0.8 pad 1.8)
  other vias: 2,42
N$4  (via drill 0.8 pad 1.8)
  other vias: 2,39
N$5  (via drill 0.8 pad 1.8)
  other vias: 2,48
N$6  (via drill 0.8 pad 1.8)
  other vias: 16,2
N$7  (via drill 0.8 pad 1.8)
  other vias: 19,2
N$8  (via drill 0.8 pad 1.8)
  other vias: 22,2
N$9  (via drill 0.8 pad 1.8)
  other vias: 86,44
N$10  (via drill 0.8 pad 1.8)
  other vias: 86,41
N$11  (via drill 1 pad 2)
  other vias: 55,75
N$12  (via drill 1 pad 2)
  other vias: 58,75
N$13  (via drill 1 pad 2)
  other vias: 61,75
N$14  (via drill 1 pad 2)
  other vias: 64,75
N$15  (via drill 1 pad 2)
  other vias: 74,2
N$16  (via drill 1 pad 2)
  other vias: 71,2
N$17  (via drill 1 pad 2)
  other vias: 68,2
N$18  (via drill 1 pad 2)
  other vias: 65,2
N$19  (via drill 0.8 pad 1.8)
  other vias: 86,38
N$20  (via drill 0.8 pad 1.8)
  other vias: 68,39
N$21  (via drill 0.8 pad 1.8)
  other vias: 68,36
N$22  (via drill 0.8 pad 1.8)
  other vias: 71,39
N$23  (via drill 0.8 pad 1.8)
  other vias: 71,36
N$24  (via drill 0.8 pad 1.8)
  other vias: 41,50
N$25  (via drill 0.8 pad 1.8)
  other vias: 44,50
N$26  (via drill 0.8 pad 1.8)
  other vias: 47,50
N$27
  Top 0.254: IC9.3 39.37,11.02 38.1,12.29 34.29,12.29 34.29,14.83 30.48,18.64 22.86,18.64 22.86,37.69 17.78,42.77 17.78,59.28 21.59,63.09 24.13,63.09 24.13,60.55 IC1.29
N$28  (1 unrouted)
N$29  (1 unrouted)
N$30  (3 unrouted)
N$31  (1 unrouted)
N$32  (2 unrouted)
N$33  (1 unrouted)
N$34  (1 unrouted)
N$35  (1 unrouted)
N$36  (1 unrouted)
N$37  (1 unrouted)
N$38  (1 unrouted)
N$39  (1 unrouted)
N$40  (1 unrouted)
N$41  (1 unrouted)
N$42  (1 unrouted)
N$43  (1 unrouted)
N$44  (1 unrouted)
N$45  (1 unrouted)
N$46  (1 unrouted)
N$47  (1 unrouted)
N$48  (1 unrouted)
N$49  (1 unrouted)
N$50  (1 unrouted)
N$51  (1 unrouted)
N$52  (1 unrouted)
N$53  (1 unrouted)
N$54  (1 unrouted)
N$55  (2 unrouted)
  Top 0.254: 33.02,30.07 33.02,27.53 U$3.P$3 | 33.02,30.07 29.21,33.88 29.21,50.39 31.75,52.93 31.75,59.28 26.67,64.36 21.59,64.36 16.51,59.28 16.51,58.01 12.7,54.2 U$2.P$4 | 33.02,30.07 U$3.P$4
N$56  (3 unrouted)
N$57  (3 unrouted)
N$58
  Top 0.254: 33.88,68.5 30.73,68.5 29.95,67.71
N$59  (1 unrouted)
N$60
  Top 0.254: C15.2 38.1,54.2 39.37,52.93 39.37,45.31 41.91,42.77 U$4.P$1
N$61  (1 unrouted)
N$62
  Top 0.254: U$4.P$2 44.45,42.77 46.99,42.77 U$4.P$3
N$63
  Top 0.254: C17.2 29.21,68.17 35.56,61.82 35.56,60.55 45.72,50.39 45.72,49.12 41.91,45.31 U$4.P$6
N$64  (1 unrouted)
N$65
  Top 0.254: C19.2 44.45,73.25 49.53,68.17 49.53,64.36 52.07,61.82 52.07,52.93 46.99,47.85 46.99,45.31 U$4.P$4
N$66  (1 unrouted)
  Top 0.254: T15.1 30.48,3.4 13.97,3.4 13.97,4.67 11.43,7.21 10.16,7.21 IC8.8
N$67  (1 unrouted)
N$69  (4 unrouted)
  Top 0.254: T6.1 52.07,19.91 50.8,18.64 43.18,18.64 43.18,22.45 38.1,27.53 35.56,27.53 35.56,33.88 31.75,37.69 31.75,51.66 33.02,52.93 33.02,59.28 27.94,64.36 27.94,70.71 29.21,71.98 29.21,73.25 34.29,73.25 34.29,71.98 T5.1
N$70
  Top 0.254: 12.32,31.9 12.32,35.78 14.99,38.45 16.69,38.45
N$71
  Top 0.254: 12.34,30.58 12.8,30.58 13.06,30.83 13.06,35.76 15.19,37.89 16.51,37.89 16.56,37.94
N$72
  Top 0.254: 12.27,29.41 12.78,29.41 13.74,30.38 13.74,35.78 15.39,37.44 16.64,37.44 16.69,37.49
N$73
  Top 0.254: 12.52,27.96 12.52,28.16 14.25,29.89 14.25,35.56 15.62,36.93 16.54,36.93 16.59,36.98
N$74  (6 unrouted)
N$75  (5 unrouted)
  Top 0.254: T2.3 40.64,31.34 52.07,31.34 52.07,33.88 T3.3
N$76
  Top 0.254: 12.04,26.79 12.27,26.79 15.06,29.59 15.06,35.66 15.8,36.4 15.82,36.4 15.95,36.52 16.54,36.52 16.56,36.55
N$77
  Top 0.254: 12.37,25.47 12.37,25.5 15.85,28.98 15.85,35.56 16.28,35.99
N$78  (3 unrouted)
  Top 0.254: T20.2 44.45,38.96 53.34,38.96 54.61,40.23 57.15,40.23 57.15,38.96 T18.2 | T15.2 33.02,3.4 36.83,3.4 38.1,2.13 40.64,2.13 40.64,4.67 43.18,4.67 T19.2
N$79
  Top 0.254: 11.94,24.33 12.39,24.33 16.87,28.8
N$80
  Top 0.254: 12.55,22.86 14.78,22.86 20.22,28.29
N$81  (2 unrouted)
  Top 0.254: T19.3 41.91,3.4 46.99,3.4 46.99,8.48 57.15,18.64 57.15,37.69 58.42,38.96 58.42,40.23 57.15,41.5 55.88,41.5 T18.3
N$82  (2 unrouted)
  Top 0.254: T19.1 43.18,2.13 63.5,2.13 63.5,7.21 77.47,21.18 77.47,24.99 81.28,28.8 81.28,35.15 83.82,37.69 83.82,44.04 86.36,46.58 86.36,55.47 69.85,71.98 55.88,71.98 54.61,73.25 45.72,73.25 45.72,75.79 38.1,75.79 38.1,70.71 30.48,70.71 30.48,71.98 T17.1
N$83
  Top 0.254: 41.3,29.59 44.35,29.59 45.34,30.58
N$84
  Top 0.254: 41.71,28.14 41.71,27.68 45.14,24.25
N$85
  Top 0.203: 32.82,41.52 32.82,37.49 34.39,35.91 34.67,35.91 34.75,35.99
N$86
  Top 0.203: 33.43,41.6 33.43,37.54 34.49,36.47 34.87,36.47
N$87
  Top 0.203: 34.06,41.52 34.06,37.54 34.62,36.98
N$88
  Top 0.203: 34.75,41.52 34.75,38.53 34.8,38.48
N$89
  Top 0.203: 58.19,28.27 58.19,27.25 61.62,23.82
N$90
  Top 0.203: 59.11,28.29 59.11,27.76 62.51,24.35
N$91
  Top 0.203: 59.99,28.27 59.99,27.66 63.25,24.41
N$92
  Top 0.203: 68.1,27.58 67.84,27.58 64.77,24.51
N$93
  Top 0.203: 68.81,27.51 68.81,27.17 68.53,26.9 68.02,26.9 65.53,24.41
N$94
  Top 0.203: 69.55,27.48 69.55,27.02 68.86,26.34 68.28,26.34 66.47,24.53
N$95
  Top 0.203: 70.18,27.58 70.18,26.77 68.81,25.4 68.25,25.4 67.28,24.43
N$96
  Top 0.203: 44.83,36.83 44.83,34.46 44.7,34.34
N$97
  Top 0.203: 42.39,37.87 42.39,35.02 42.98,34.44
N$98
  Top 0.203: 35.84,34.72 35.84,34.36 36.45,33.75 36.45,30.88 37.77,29.56
N$99
  Top 0.203: 38.3,34.87 38.3,34.31 41.4,31.21
N$100
  Top 0.203: 37.9,34.82 37.9,33.24 40.54,30.6 40.54,30.48 41.38,29.64
N$101
  Top 0.203: 37.31,34.79 37.31,33.14 39.88,30.58 39.88,29.49 41.12,28.24
N$102
  Top 0.203: 24.08,12.72 27.38,12.72 32.05,8.05
N$103
  Top 0.203: 24.33,10.26 28.07,10.26 30.45,7.87
N$104
  Top 0.203: 24.03,10.03 24.16,10.03 26.26,7.92 26.26,6.98 24.87,5.58
N$105
  Top 0.203: 21.51,11.43 21.51,6.83 22.89,5.46
N$106
  Top 0.203: 16.03,11.12 17.45,11.12 20.3,13.97 23.06,13.97 24.11,12.92
N$107
  Top 0.203: 16.05,9.88 17.42,9.88 20.52,12.98 21.26,12.98 22.45,11.78
N$108
  Top 0.203: 12.19,2.08 12.19,1.75 12.88,1.06 15.09,1.06 15.95,1.93
N$109
  Top 0.203: 11.68,2.03 11.68,1.65 12.75,0.58 17.8,0.58 18.9,1.67
N$110
  Top 0.203: 22.68,1.72 29.06,1.72 30.79,3.45
N$111
  Top 0.203: 2.97,5.3 2.97,11.63 4.17,12.82
N$112
  Top 0.203: 4.37,14.63 5.36,14.63 6.25,13.74 6.25,5.41 6.45,5.2
N$113
  Top 0.203: 5.26,22.93 5.26,22.48 9.5,18.23
N$114
  Top 0.203: 5.33,25.45 3.66,25.45 2.34,24.13 2.34,16.3 3.99,14.65
N$115
  Top 0.203: 5.16,31.77 7.67,31.77 11.68,35.78
N$116
  Top 0.203: 9.7,36.42 7.42,36.42 3.71,32.71 3.71,32.08 3.86,31.92 5.82,31.92 5.84,31.95
N$117
  Top 0.203: 10.54,39.16 6.88,39.16 5.77,38.05
N$118
  Top 0.203: 2.06,35.81 2.06,34.84 3.02,33.88 3.02,31.49 3.79,30.73 5.77,30.73 5.84,30.65
N$119
  Top 0.203: 1.63,38.55 1.42,38.55 0.56,37.69 0.56,32.13 3.23,29.46 6.15,29.46 6.25,29.56
N$120
  Top 0.203: 2.23,41.58 3.58,41.58 5.44,39.72
N$121
  Top 0.203: 14.43,43.48 16.26,43.48 19.99,39.75
N$122
  Top 0.203: 13.13,43.18 13.13,42.8 13.21,42.72 16.43,42.72 19.41,39.75 19.41,39.47 19.43,39.44
N$123
  Top 0.203: 11.73,43.28 11.73,43.08 12.62,42.19 16.43,42.19 18.95,39.67
N$124
  Top 0.203: 10.62,43.28 10.74,43.28 12.45,41.58 16.54,41.58 18.52,39.59
N$125
  Top 0.203: 9.14,43.18 9.37,43.18 11.86,40.69 16.89,40.69 17.91,39.67
N$126
  Top 0.203: 8,43.2 8.2,43.2 11.68,39.72 17.32,39.72 17.5,39.54
N$127
  Top 0.203: 6.6,43.05 6.93,43.05 10.57,39.42
N$128
  Top 0.203: 5.41,43.53 5.41,39.7 5.44,39.67
N$129
  Top 0.203: 8.43,47.62 8.43,48.51 7.95,48.99
N$130
  Top 0.203: 8.94,47.62 8.94,48.54 9.37,48.97
N$131
  Top 0.203: 9.42,47.72 9.42,47.8 10.39,48.76
N$132
  Top 0.203: 9.98,47.57 10.57,47.57 11.91,48.92
N$133
  Top 0.203: 10.06,46.83 11.25,46.83 13.16,48.74
N$134
  Top 0.203: 11.4,46.78 13.31,44.88
N$135
  Top 0.203: 9.96,46.15 10.77,46.15 12.01,44.9
N$136
  Top 0.203: 9.47,46.15 9.47,45.69 9.68,45.49 10.19,45.49 10.72,44.95
N$137
  Top 0.203: 8.99,46.12 8.99,44.98 9.45,44.52
N$138
  Top 0.203: 8.46,46.07 8.46,45.23 7.98,44.75
N$139
  Top 0.203: 8.05,46.89 8.05,46.2 6.68,44.83
N$140
  Top 0.203: 8.15,46.89 7.47,46.89 6.73,47.62 6.73,49.4 6.76,49.42
N$141
  Top 0.203: 23.14,44.9 21.03,44.9 21.01,44.88
N$142
  Top 0.203: 23.32,43.41 20.8,43.41 20.73,43.48
N$143
  Top 0.203: 24.64,44.9 24.64,45.77 25.07,46.2 27.13,46.2
N$144
  Top 0.203: 24.64,43.41 24.64,42.52 25.43,41.73 27.23,41.73
N$145
  Top 0.203: 24.64,44.47 26.82,44.47 26.92,44.37
N$146
  Top 0.203: 24.69,43.94 26.9,43.94 27,43.84
N$147
  Top 0.203: 23.95,45.23 23.95,47.42 24.36,47.83 25.45,47.83 26.49,46.78
N$148
  Top 0.203: 23.77,43.08 23.77,42.16 24.79,41.14 26.98,41.14 27.1,41.27
N$149
  Top 0.203: 27.51,49.63 27.51,49.37 28.55,48.33 28.55,42.72 27.89,42.06
N$150
  Top 0.203: 24.87,49.32 24.87,48.81 25.15,48.54 25.96,48.54 27.79,46.71
N$151
  Top 0.203: 21.67,49.27 21.67,47.37 20.02,45.72
N$152
  Top 0.203: 22.58,49.27 22.58,45.39 23.09,44.88
N$153
  Top 0.203: 23.27,49.6 23.27,45.69 23.9,45.06
N$154
  Top 0.203: 24.26,51.61 24.26,54.86 24.31,54.91
N$155
  Top 0.203: 26.14,56.59 26.64,56.59 28.42,58.37
N$156
  Top 0.203: 26.06,54.68 26.29,54.68 28.47,52.5
N$157
  Top 0.203: 26.24,56.03 27.74,56.03 28.5,56.79
N$158
  Top 0.203: 26.24,55.04 27.64,55.04 28.4,54.28
N$159
  Top 0.203: 26.19,55.57 27.99,55.57 28.5,55.06
N$160
  Top 0.203: 22.66,56.66 22.66,57.2 23.42,57.96 26.04,57.96 27.36,59.28
N$161
  Top 0.203: 22.71,56.08 22.58,56.08 22.02,56.64 22.02,57.17 23.22,58.37 25.55,58.37 26.57,59.38
N$162
  Top 0.203: 22.68,54.58 22.25,54.58 22.05,54.38 22.05,53.69 23.32,52.42 23.32,51.51 23.24,51.43
N$163
  Top 0.203: 22.58,55.11 22.1,55.11 21.46,54.48 21.46,53.44 22.5,52.4 22.5,51.28
N$164
  Top 0.203: 22.71,55.57 21.72,55.57 21.39,55.9 20.4,55.9
N$165
  Top 0.203: 2.06,56.08 7.24,56.08 10.21,59.05
N$166
  Top 0.203: 12.95,53.69 13.92,53.69 14.94,52.68 14.94,50.44 14.35,49.86
N$167
  Top 0.203: 12.29,58.85 11.86,58.85 11.38,58.37 11.38,52.4 13.21,50.57
N$168
  Top 0.203: 9.8,56.44 9.8,55.78 7.92,53.89 7.92,52.78 5.59,50.44
N$169
  Top 0.203: 9.93,53.95 9.93,52.37 7.95,50.39
N$170
  Top 0.203: 13.01,67.56 9.96,67.56 9.14,68.37
N$171
  Top 0.203: 8.99,65.88 11.79,65.88 13.31,64.36
N$172
  Top 0.203: 7.54,67.15 4.98,67.15 3.79,68.35
N$173
  Top 0.203: 7.72,65.83 5.16,65.83 3.86,64.54
N$174
  Top 0.203: 2.06,67.1 1.8,67.1 0.69,65.99 0.69,63.93 2.59,62.02
N$175
  Top 0.203: 2.95,64.56 2.95,64.33 4.34,62.94 4.34,61.67 3.23,60.55
N$176
  Top 0.203: 3,68.42 3,73.15 4.14,74.29
N$177
  Top 0.203: 7.82,74.11 13.21,74.11 13.69,74.6
N$178
  Top 0.203: 7.29,72.49 13.31,72.49 13.79,72
N$179
  Top 0.203: 14.73,67.66 14.73,69.26 16.99,71.52
N$180
  Top 0.203: 14.73,64.84 15.27,64.84 19.61,69.19 19.61,71.32 19.36,71.57
N$181
  Top 0.203: 21.61,66.67 21.61,71.17 21.79,71.34
N$182
  Top 0.203: 24.41,67.28 24.41,71.37 24.33,71.45
N$183
  Top 0.203: 28.52,76.4 25.76,76.4 24.51,75.16
N$184
  Top 0.203: 28.42,73.2 25.93,73.2 25.04,72.31
N$185
  Top 0.203: 30.91,74.44 30.91,76.02 30.48,76.45
N$186
  Top 0.203: 30.63,76.25 35.26,76.25 35.81,75.69
N$187
  Top 0.203: 35.97,72.77 35.97,74.57 36.07,74.67
N$188
  Top 0.203: 29.82,65.05 29.82,64.69 34.24,60.27 34.24,56.56 35.87,54.94
N$189
  Top 0.203: 61.06,48.36 61.06,52.32 62.1,53.36
N$190
  Top 0.203: 62.15,55.24 60.55,55.24 58.83,53.51 58.83,48.76 58.55,48.48
N$191
  Top 0.203: 67.92,47.83 70,47.83 73.28,51.1
N$192
  Top 0.203: 76.22,51.3 76.22,51.76 80.44,55.98 83.01,55.98 85.04,53.95
N$193
  Top 0.203: 76.2,48.71 76.2,49.35 78.94,52.09 78.94,52.98 80.95,54.99 82.73,54.99 83.82,53.89
N$194
  Top 0.203: 76.48,45.82 76.48,43.66 74.19,41.37
N$195
  Top 0.203: 73.03,45.94 70.31,45.94 67.69,43.33
N$196
  Top 0.203: 73.28,48.48 73.79,48.48 74.7,47.57 74.7,44.55 73.28,43.13 73,43.13 72.47,42.59 72.47,41.63 72.62,41.48
N$197
  Top 0.203: 67.18,55.32 73.25,55.32 75.62,57.68
N$198
  Top 0.203: 67.36,53.06 75.36,53.06 79.91,57.6
N$199
  Top 0.203: 78.99,66.98 81.48,66.98 84.3,64.16
N$200
  Top 0.203: 77.27,66.34 77.27,66.27 80.47,63.06 81.81,63.06 81.97,62.91
N$201
  Top 0.203: 78.44,69.87 82.07,69.87 86.64,65.3 86.64,63.24 84.63,61.24
N$202
  Top 0.203: 77.85,75.33 81.74,75.33 82.53,74.55
N$203
  Top 0.203: 86.36,75.56 86.36,76.53 85.83,77.06 76.25,77.06 75.74,76.55 75.74,76.09 75.79,76.04
N$204
  Top 0.203: 86.33,74.01 85.9,74.01 84.18,72.28 80.11,72.28 78.56,73.83 78.08,73.83
N$205
  Top 0.203: 86.23,72.44 86.23,72.23 85.01,71.02 78.74,71.02 77.55,72.21 77.55,72.79 77.27,73.07
N$206
  Top 0.203: 76.81,73.07 76.81,72.13 78,70.94 78,70.13 77.98,70.1
N$207
  Top 0.203: 76.3,73.1 76.3,69.9 79.2,67
N$208
  Top 0.203: 75.06,73.91 74.52,73.91 73.58,72.97 73.58,70.41 77.24,66.75
N$209
  Top 0.203: 70.81,74.04 73.48,74.04 74.88,75.43
N$210
  Top 0.203: 67.82,74.11 65.61,74.11 64.67,75.05
N$211
  Top 0.203: 54.23,75.16 52.93,75.16 52.3,75.79
N$212
  Top 0.203: 47.19,75.18 48.87,75.18 50.24,73.81
N$213
  Top 0.203: 47.65,76.32 48.39,76.32 49.58,77.52 58.98,77.52 61.16,75.33
N$214
  Top 0.203: 57.76,74.62 58.04,74.62 59.46,73.2 62.48,73.2 64.01,74.72
N$215
  Top 0.203: 46.71,64.74 49.23,62.23
N$216
  Top 0.203: 45.74,68.65 45.74,69.57 41.88,73.43
N$217
  Top 0.203: 47.45,58.52 47.42,58.52 46.05,57.15 46.05,56.51
N$218
  Top 0.203: 50.44,58.47 50.44,53.69 49.68,52.93
N$219
  Top 0.203: 45.01,54.91 44.48,54.91 43.71,55.67 43.71,64.36 44.58,65.22
N$220
  Top 0.203: 54.99,64.87 57.38,64.87 61.01,61.24
N$221
  Top 0.203: 62.61,61.44 63.02,61.44 64.59,59.86
N$222
  Top 0.203: 66.67,60.91 66.67,63.57 64.41,65.83
N$223
  Top 0.203: 73.33,62.89 73.33,61.82 70.69,59.18 66.9,59.18 66.78,59.05
N$224
  Top 0.203: 58.27,60.09 61.67,60.09 62.79,61.21
N$225
  Top 0.203: 58.12,58.06 62.92,58.06 64.59,59.74
N$226
  Top 0.203: 54.66,60.12 54.66,64.77 54.76,64.87
N$227
  Top 0.203: 54.69,59.64 54.46,59.64 53.98,60.12 53.98,64.44 53.52,64.89
N$228
  Top 0.203: 52.27,64.64 52.65,64.64 53.29,64 53.29,60.19 54.25,59.23 54.48,59.23 54.59,59.13
N$229
  Top 0.203: 54.74,58.62 54.13,58.62 52.81,59.94 52.81,63.01 51.08,64.74
N$230
  Top 0.203: 56.31,50.75 58.55,48.51
N$231
  Top 0.203: 54.71,58.19 54.53,58.19 53.47,57.12 53.47,54.76 54.43,53.79
N$232
  Top 0.203: 58.14,58.09 58.14,55.8 56.26,53.92
N$233  (1 unrouted)
  Top 0.203: 35.51,49.81 35.51,49.78
N$234
  Top 0.203: 37.62,49.88 37.62,53.44 38.51,54.33
N$235
  Top 0.203: 35.69,49.48 35.69,47.27 34.82,46.4
N$236
  Top 0.203: 36.07,54.28 36.07,50.59 35.36,49.88
N$237
  Top 0.203: 30.45,47.14 31.67,47.14 31.7,47.16
N$238
  Top 0.203: 30.43,45.51 31.57,45.51 31.67,45.61
N$239
  Top 0.203: 53.01,30.4 53.01,32.48 52.15,33.35
N$240
  Top 0.203: 54.23,29.1 54.23,24.63
N$241
  Top 0.203: 52.91,23.64 52.91,21.2 52.3,20.6
N$242
  Top 0.203: 50.44,23.67 50.44,20.95 50.8,20.6
N$243
  Top 0.203: 47.98,23.64 47.98,21.69 49.2,20.47
N$244
  Top 0.203: 74.47,41.37 74.47,39.59 73.64,38.76 71.42,38.76 71.37,38.81
N$245
  Top 0.203: 71.42,35.94 73.43,35.94 74.78,34.59
N$246
  Top 0.203: 68.61,39.34 68.61,40.08 69.55,41.02 72.16,41.02 72.64,41.5
N$247
  Top 0.203: 67.94,35.73 65.1,35.73 64.87,35.96
N$248
  Top 0.203: 63.91,39.19 63.91,39.47 67.67,43.23
N$249
  Top 0.203: 64.95,38.38 67.31,38.38 68,39.06
N$250
  Top 0.203: 60.91,48.59 62.23,48.59 63.93,46.89
N$251
  Top 0.203: 63.98,39.52 63.98,46.81 63.86,46.94
N$252
  Top 0.203: 53.95,46.28 55.68,46.28 58.27,43.68
N$253
  Top 0.203: 53.42,44.34 53.42,43.08 54.08,42.41 55.55,42.41 56.49,43.35
N$254
  Top 0.203: 51.94,44.12 51.94,43.25 53.72,41.48 55.8,41.48 55.83,41.5
N$255
  Top 0.203: 51.26,45.36 50.72,45.36 50.39,45.03 50.39,41.04 49.28,39.92 45.57,39.92 44.68,39.04
N$256
  Top 0.381: 85.34,19.94 85.34,18.82 87.25,16.91 87.25,7.46 84.86,5.08
N$257
  Top 0.381: 79.3,21.59 79.3,17.88 77.17,15.74
N$258
  Top 0.381: 74.27,15.26 74.27,9.77 74.42,9.62
N$259
  Top 0.381: 68.4,7.74 68.61,7.74 71.63,10.77 72.97,10.77 73.97,9.77
N$260
  Top 0.381: 68.48,5.79 72.24,5.79 72.72,6.27
N$261
  Top 0.381: 76.07,4.44 75.87,4.44 74.32,5.99
N$262
  Top 0.381: 76.07,6.19 76.43,6.19 77.85,4.77
N$263
  Top 0.381: 74.6,10.08 80.77,10.08 81.31,10.61
N$264
  Top 0.381: 81.28,15.67 77.47,15.67 77.42,15.62
N$265
  Top 0.381: 55.32,8.68 57.71,8.68 59.44,6.96
N$266
  Top 0.381: 55.24,7.34 55.24,6.85 58.34,3.76
N$267
  Top 0.381: 51.99,4.19 52.55,4.19 55.32,6.96
N$268
  Top 0.381: 51.46,6.73 51.46,7.23 54.99,10.77
N$269
  Top 0.381: 49.76,5.58 49.76,8.45 54.13,12.82
N$270
  Top 0.381: 56.13,12.77 56.13,13 58.57,15.44
N$271
  Top 0.381: 59.38,7.23 61.67,7.23 66.55,12.11
N$272
  Top 0.381: 69.9,21.23 69.9,23.01 74.68,27.78
N$273
  Top 0.381: 70.1,20.39 70.99,20.39 72.24,21.64 72.24,23.85 76.05,27.66
N$274
  Top 0.381: 77.32,27.78 77.32,27.02 75.77,25.47 75.77,23.87 70.54,18.64
N$275
  Top 0.381: 41.58,49.98 43.43,49.98 43.51,49.91
N$276
  Top 0.254: 47.17,51.91 47.17,50.75 46.99,50.57
N$277
  Top 0.254: 37.64,60.88 37.64,62.38 35.53,64.49 35.53,64.92 35.51,64.94
N$278
  Top 0.254: 40.28,59.48 41.5,59.48 42.44,60.42 42.44,64.72 38.63,68.53
N$279
  Top 0.254: 38.43,65.94 38.43,63.11 39.24,62.3
N$280
  Top 0.254: 37.59,69.16 40.66,69.16 44.58,65.25
N$281
  Top 0.254: 36.98,69.62 36.98,69.8 37.19,70 44.15,70 45.77,68.37
N$282
  Top 0.254: 35.03,69.62 30.23,69.62 29.87,69.97 29.87,71.88 30.28,72.28
N$283
  Top 0.254: 8.87,64.33 8.87,60.19 10.26,58.8
N$284
  Top 0.254: 4.57,72.26 4.57,71.88 8.1,68.35
N$285
  Top 0.254: 20.04,34.92 20.04,29.28 19.94,29.18
N$286
  Top 0.254: 20.73,35.94 20.73,30.68 21.89,29.51 21.89,24.46 21.06,23.62
N$287
  Top 0.254: 14.17,18.59 19.36,18.59 20.6,19.83
N$288
  Top 0.254: 27.58,19.71 30.12,19.71 32.82,17.01 36.22,17.01 36.55,16.68
N$289
  Top 0.254: 27.48,23.06 28.75,23.06 33.83,17.98 35.87,17.98 36.6,17.24
N$290
  Top 0.254: 16.13,7.31 18.95,7.31 20.85,5.41 23.27,5.41 23.32,5.36
N$291
  Top 0.254: 10.64,9.98 13.34,9.98 14.63,11.27
N$292
  Top 0.254: 10.85,8.61 13.69,8.61 14.91,7.39
N$293
  Top 0.254: 28.32,26.74 28.32,26.46 34.87,19.91 38.38,19.91 40.44,21.97
N$294
  Top 0.254: 30.79,27.05 31.24,27.05 35.56,22.73
N$295
  Top 0.254: 28.17,29.94 28.14,29.94 25.35,32.74 25.35,34.13 25.32,34.16
N$296
  Top 0.254: 28.4,34.19 28.4,32.36 30.66,30.09
N$297
  Top 0.254: 28.5,36.17 28.5,40.84 27.79,41.55
N$298
  Top 0.254: 51.08,37 53.21,37 55.17,38.96
N$299
  Top 0.254: 60.12,31.44 66.9,31.44 68.05,32.59
N$300
  Top 0.254: 60.07,28.83 67.41,28.83 68.17,28.06
N$301
  Top 0.254: 85.17,25.09 85.17,27.71 82.88,29.99 82.88,32.23 82.86,32.25
N$302
  Top 0.254: 86.41,22.42 86.69,22.42 87.27,23.01 87.27,25.37 86.54,26.11 86.54,30.27 84.89,31.92
N$303
  Top 0.254: 85.29,44.04 85.27,44.04 84.56,43.33 84.56,41.75 85.57,40.74
N$304
  Top 0.254: 85.45,37.74 85.24,37.74 83.36,35.86 83.36,35.56 83.34,35.53
N$305
  Top 0.508: 1.98,51.76 1.98,50.42 4.09,48.31 4.09,46.76 2.23,44.9
N$306
  Top 0.508: 19.89,27.94 19.89,24.91 13.92,18.95
N$307
  Top 0.508: 63.96,70.38 66.88,70.38 68.15,69.11 68.15,68.19 68.2,68.14 63.63,68.14 63.58,68.19
N$308
  Top 0.508: 46.89,14.55 48.39,14.55 50.6,16.76
N$309
  Top 0.508: 59.44,7.36 59.44,10.89 61.62,13.08
N$310
  Top 0.508: 62.61,53.29 62.61,51.94 66.6,47.95
N$311
  Top 0.508: 66.93,58.77 66.93,58.72 68.56,57.1 75.23,57.1 75.89,57.76
N$312
  Top 0.508: 68.3,68.22 68.3,62.23 66.83,60.75
N$313
  Top 0.508: 38.68,54.86 39.65,54.86 43.87,50.64
N$314
  Top 0.508: 4.37,14.83 4.37,15.31 7.26,18.21 10.59,18.21 10.82,18.44
N$315
  Top 0.508: 31.77,5.79 38.35,5.79 38.41,5.74
N$316
  Top 0.508: 39.14,3.88 39.14,4.19 40.49,5.53 44.35,5.53 45.67,6.85 45.67,10.33 45.92,10.59
N$317
  Top 0.508: 74.17,1.88 81.41,1.88 84.51,4.98
N$318
  Top 0.508: 71.14,2.77 71.14,2.79 74.35,5.99
N$319
  Top 0.508: 68.22,2.21 68.22,5.46 68.58,5.81
N$320
  Top 0.508: 64.92,2.51 64.92,4.95 67.87,7.9
N$321
  Top 0.508: 81.25,13.23 79.12,13.23 77.44,14.91
N$322
  Top 0.508: 84.12,16.23 84.12,17.4 82.63,18.89 82.63,19.91 85.34,22.63
N$323
  Top 0.508: 79.35,22.78 79.35,24.15 82.12,26.92 83.64,26.92 85.78,24.79
N$324
  Top 0.508: 26.87,36.19 26.87,41.65 26.72,41.8
N$325
  Top 0.254: 37.36,49.35 37.36,40.74 36.4,39.77
N$326
  Top 0.254: 42.06,42.82 40.51,42.82 37.31,39.62
N$327
  Top 0.254: 44.53,42.57 43.69,42.57 42.75,41.63 40.46,41.63 38.38,39.54
N$328
  Top 0.254: 44.78,36.93 49.84,36.93 50.04,37.13
N$329
  Top 0.254: 18.64,52.47 18.64,43.91 19.89,42.67
N$330
  Top 0.254: 54.2,23.59 54.2,19.88 51.18,16.86
N$331
  Top 0.254: 13.21,58.92 13.21,59.48 20.95,67.23
N$332
  Top 0.254: 12.93,56.46 12.93,57.32 20.4,64.79 20.47,64.79 20.88,65.2 23.14,65.2 24.21,66.27
N$333
  Top 0.254: 49.05,58.95 49.05,59.03 47.12,60.96 47.12,64.33 46.66,64.79
N$334
  Top 0.254: 50.34,73.71 50.34,71.85 51.03,71.17
N$335
  Top 0.254: 52.15,74.95 52.15,71.67 52.27,71.55
N$336
  Top 0.254: 54.97,71.5 55.65,71.5 57.76,69.39
N$337
  Top 0.254: 53.52,70.18 53.52,68.78 50.8,66.06
N$338
  Top 0.254: 58.83,47.9 58.83,46.43 61.49,43.76 61.49,39.59 61.54,39.54
N$339
  Top 0.254: 62.53,39.54 62.53,44.09 60.81,45.82 60.81,48.05 60.55,48.31
N$340
  Top 0.254: 64.95,37.46 65.73,37.46 66.12,37.84 69.9,37.84 70.64,38.58
N$341
  Top 0.254: 65.13,36.98 66.73,36.98 66.95,37.21 70,37.21 70.66,36.55
N$342
  Top 0.254: 81.13,47.04 81.1,47.04 78.11,44.04 78.11,35.15 78.59,34.67
N$343
  Top 0.254: 86.44,40.53 86.44,40.13 87.22,39.34 87.22,36.42 86.06,35.25 84.91,35.25 84.86,35.3
N$344
  Top 0.254: 83.8,43 82.17,43 82.12,42.95
N$345
  Top 0.254: 80.64,37.97 80.64,30.02 78.87,28.24
N$346
  Top 0.254: 45.31,28.98 45.31,26.26 46.76,24.81
N$347
  Top 0.254: 52.98,29.1 52.98,27.71 50.24,24.97
N$348
  Top 0.254: 49.1,28.98 49.1,24.86 49.33,24.63
N$349
  Top 0.254: 46.66,29.1 46.66,26.34 47.9,25.09
N$350
  Top 0.254: 27.38,60.96 28.45,60.96 30.38,59.03 30.38,58.42 30.25,58.29
N$351
  Top 0.254: 29.82,52.45 29.82,52.4 27.43,50.01
N$352
  Top 0.254: 15.21,74.57 16.1,74.57 16.15,74.62
N$353
  Top 0.254: 17.65,74.57 18.57,74.57 18.62,74.62
N$354
  Top 0.254: 22.68,74.55 23.62,74.55 23.67,74.6
N$355
  Top 0.254: 20.12,74.7 21.08,74.7 21.11,74.72
N$356
  Top 0.254: 21.92,73.89 21.92,72.87
N$357
  Top 0.254: 24.46,72.87 24.46,73.96
N$358
  Top 0.254: 74.32,64.46 75.79,64.46 80.37,59.89 80.37,57.45 80.44,57.38
N$359
  Top 0.254: 74.37,64 74.37,60.14 76.5,58.01
N$360
  Top 0.254: 66.98,60.68 68.58,60.68 70.81,62.91
N$361
  Top 0.254: 67.03,70.43 69.29,70.43 71.75,67.97 71.75,67.59 71.86,67.48
N$362
  Top 0.203: 60.94,69.03 61.75,69.03 63.27,70.56
N$363
  Top 0.203: 61.19,67.51 61.82,67.51 63.07,66.27
N$364
  Top 0.203: 61.16,68.07 63.04,68.07 63.2,68.22
N$365
  Top 0.203: 61.19,68.55 63.52,68.55
N$366
  Top 0.203: 59.89,69.11 59.89,69.97 60.63,70.71 63.3,70.71 63.42,70.58
N$367
  Top 0.203: 59.87,67.51 59.87,66.34 58.95,65.43 55.37,65.43 54.94,65.86
N$368
  Top 0.203: 40.11,58.77 40.11,56.99 45.41,51.69 45.9,51.69 46.1,51.89
N$369
  Top 0.203: 49.71,55.52 49.71,57.7 49.1,58.31
N$370
  Top 0.203: 55.3,50.59 55.3,49.07 60.53,43.84 60.53,38.48
N$371
  Top 0.203: 63.73,19.76 63.73,19.96 61.54,22.15
N$372
  Top 0.203: 62.48,22.2 62.48,21.69 64.21,19.96 64.21,19.68
N$373
  Top 0.203: 63.3,22.15 63.3,21.46 64.75,20.01 64.75,19.78
N$374
  Top 0.203: 65.89,19 66.14,19 68.38,21.23
N$375
  Top 0.203: 65.86,17.52 66.27,17.52 68.33,15.47
N$376
  Top 0.203: 63.86,16.81 63.86,16.15 62.33,14.63
N$377
  Top 0.203: 65.18,16.81 65.18,16.48 67.28,14.37
N$378
  Top 0.203: 64.72,16.73 64.72,15.54 65.71,14.55
N$379
  Top 0.203: 64.26,16.68 64.26,14.8 63.93,14.47
N$380
  Top 0.203: 63.07,17.57 61.77,17.57 60.45,16.25
N$381
  Top 0.203: 63.02,19 62.79,19 60.63,21.16
N$382
  Top 0.203: 63.04,18.54 61.59,18.54 60.6,19.53
N$383
  Top 0.203: 62.99,18.03 60.45,18.03 60.33,17.9
N$384
  Top 0.203: 65.2,19.83 65.2,20.82 66.47,22.09
N$385
  Top 0.203: 65.96,18.51 67.23,18.51 68.28,19.55
N$386
  Top 0.203: 65.94,18.01 67.28,18.01 68.35,16.94
N$387
  Top 0.203: 56.36,12.65 56.77,12.65 59.41,10
N$388
  Top 0.203: 33.63,26.97 35.36,26.97 39.5,22.83
N$389
  Top 0.203: 45.09,45.59 45.09,47.44 47.12,49.48
N$390
  Top 0.203: 49.17,61.82 49.4,61.82 51.46,59.76 51.46,53.64 49.89,52.07 48.82,52.07 48.74,51.99
N$391
  Top 0.203: 63.96,24.25 63.96,28.72 63.93,28.75
N$392
  Top 0.203: 25.98,54.38 25.98,53.18 27.46,51.71
N$393
  Top 0.203: 24.77,54.56 24.77,52.8 25.91,51.66
N$394
  Top 0.203: 6.55,24.2 8.31,24.2 8.43,24.33 8.43,29.59 10.9,32.05
N$395
  Top 0.203: 10.82,29.26 9.93,29.26 9.7,29.03 9.7,23.9 10.72,22.88
N$396
  Top 0.203: 2.54,38.78 4.5,38.78 5.33,37.94
N$397
  Top 0.203: 62.79,55.27 64.64,55.27 66.73,53.18
N$398
  Top 0.203: 64.67,59.53 64.67,56.38 66.47,54.58
N$399
  Top 0.203: 66.65,58.8 66.65,55.62 66.98,55.29
N$400
  Top 0.203: 64.11,34.74 65.61,34.74 65.94,34.41 69.6,34.41 70.84,35.66
N$401
  Top 0.203: 60.53,67.03 60.53,63.78 62.76,61.54
N$402
  Top 0.203: 26.06,23.67 25.07,23.67 23.8,22.4 23.8,20.24 24.33,19.71 26.36,19.71 26.42,19.76
N$403
  Top 0.203: 17.4,34.9 17.4,29 17.07,28.67
N$404
  Top 0.203: 18.9,34.82 18.9,30.12 20.14,28.88
N$405
  Top 0.203: 11.66,22.86 11.66,20.95 13.56,19.05
N$406
  Top 0.203: 30.12,7.74 30.12,7.01 31.62,5.51
N$407
  Top 0.203: 48.92,33.07 48.92,32.84 49.71,32.05 50.24,32.05 50.55,32.36 50.55,33.27 50.6,33.32
N$408
  Top 0.203: 67,53.29 67,51.91 67.72,51.2 73.1,51.2 73.15,51.15
N$409
  Top 0.203: 62.87,53.92 64.16,53.92 67.59,50.49 72.54,50.49 73.03,50.97
N$410
  Top 0.203: 62.26,54.58 61.39,54.58 59.77,52.95 59.77,49.7 60.53,48.94
N$411
  Top 0.203: 68.86,32.18 68.86,28.98 69.44,28.39
N$412
  Top 0.203: 70.18,32.18 73.79,32.18 74.88,33.27
N$413
  Top 0.203: 69.49,32.05 69.49,31.37 70.13,30.73 74.37,30.73 75.72,32.08
N$414
  Top 0.203: 70.18,28.34 70.18,29.56 70.79,30.17 75.06,30.17 76.07,29.16
N$415
  Top 0.203: 59.11,29.13 59.11,29.64 59.41,29.94 66.85,29.94 68.83,31.92
N$416
  Top 0.203: 58.06,29.38 58.06,29.54 59.87,31.34
N$417
  Top 0.203: 60.38,35.91 60.63,35.91 61.47,35.07
N$418
  Top 0.203: 50.47,29.03 50.47,27.55 51.18,27.55 51.79,28.16 51.79,29.56 51.71,29.64
N$419
  Top 0.203: 51.84,47.09 51.84,47.85 52.43,47.85 52.43,47.09 52.38,47.04
N$420
  Top 0.203: 44.98,53.46 41.66,56.79 41.66,57.63 39.98,59.31
N$421
  Top 0.203: 44.93,64.69 44.93,61.31 47.52,58.72
N$422
  Top 0.203: 47.17,56.61 47.17,57.96 47.57,58.37
N$423
  Top 0.203: 48.03,56.61 48.03,57.58 48.9,58.44
N$424
  Top 0.203: 74.27,6.8 74.27,7.16 75.03,7.92 81,7.92 81.08,8
N$425
  Top 0.203: 84.94,13.2 85.47,13.2 86.08,12.59 86.08,11.71 84.96,10.59
N$426
  Top 0.203: 83.95,7.67 83.95,7.64 82.25,5.94
N$427
  Top 0.203: 3,52 2.45,52 2.26,52.19 2.26,51.99 2.34,51.91 3.1,51.91 5.54,49.48
N$428
  Top 0.203: 36.47,14.3 36.47,15.36 35.84,16
N$429
  Top 0.203: 38.02,14.32 38.02,15.11 38.89,15.97
V+  (3 unrouted)
  Top 0.203: 52.05,51.64 52.05,51.66 54.33,53.95
  Top 0.254: 60.96,33.88 58.42,31.34 U10.5 | 74.93,33.88 60.96,33.88 | 74.93,33.88 74.93,35.15 77.47,37.69 77.47,49.12 81.28,52.93 IC14.8 | 74.93,33.88 IC13.8 | U8.5 3.81,3.4 5.08,2.13 7.62,2.13 7.62,11.02 11.43,14.83 33.02,14.83 33.02,9.75 35.56,7.21 44.45,7.21 44.45,12.29 49.53,12.29 55.88,18.64 55.88,31.34 52.07,35.15 45.72,35.15 45.72,33.88 44.45,32.61 40.64,32.61 40.64,37.69 44.45,41.5 49.53,41.5 49.53,49.12 52.05,51.64 52.07,51.66 59.69,44.04 59.69,35.15 60.96,33.88
V-  (4 unrouted)
  Top 0.254: IC13.4 78.74,28.8 80.01,30.07 80.01,36.42 78.74,37.69 78.74,42.77 81.28,45.31 83.82,45.31 85.09,46.58 IC14.4

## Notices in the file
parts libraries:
SparkFun-AnalogIC: Licensing:Creative Commons ShareAlike 4.0 International - https://creativecommons.org/licenses/by-sa/4.0
